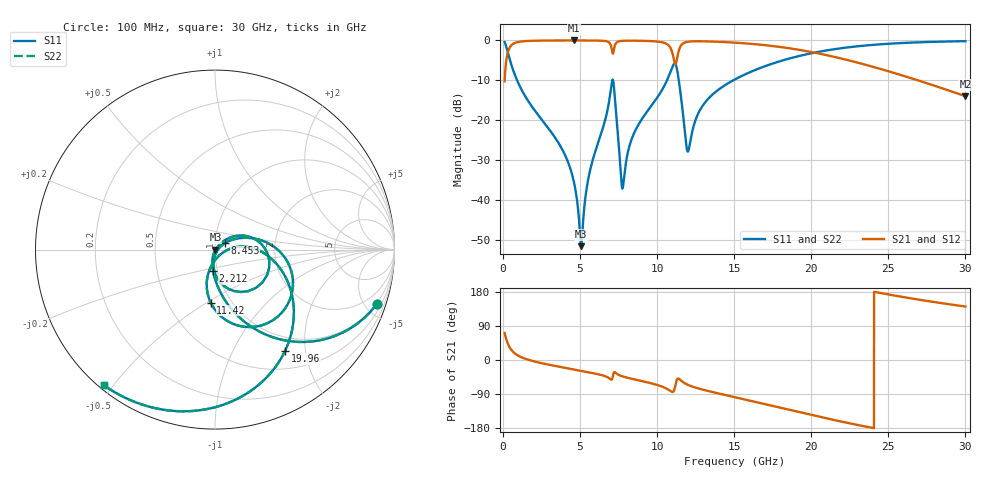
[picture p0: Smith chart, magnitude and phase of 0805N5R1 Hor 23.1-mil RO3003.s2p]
# GHz S MA R 50
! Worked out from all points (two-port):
!   3201 points, 100 MHz to 30 GHz, reference 50 ohm
!   highest |S21| = -0.02 dB at 4.594 GHz (marker M1); lowest = -14.0 dB at 30 GHz (marker M2)
!   |S21| within 3 dB of the highest: 307.7 MHz to 7.094 GHz (6.786 GHz wide, 183 % of centre); 11.37 GHz to 20.14 GHz (8.769 GHz wide, 55.7 % of centre)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
!   lowest |S11| = -51.5 dB at 5.071 GHz (marker M3), VSWR 1.01, Z = 50.2 - j0.12 ohm
!   |S11| at or under -10 dB: 908.1 MHz to 7.086 GHz (6.178 GHz wide, 155 % of centre); 7.138 GHz to 10.64 GHz (3.499 GHz wide, 39.4 % of centre); 11.4 GHz to 14.94 GHz (3.533 GHz wide, 26.8 % of centre)
!   |S22| runs from -51.5 to -0.2 dB; largest |S21 - S12| = 0
!   S11 on the Smith chart (normalised r, x): 100 MHz: 0.94, -6.00; 2.212 GHz: 0.95, -0.23; 8.453 GHz: 1.11, +0.08; 11.42 GHz: 0.80, -0.52; 19.96 GHz: 0.77, -1.64; 30 GHz: 0.01, -0.47
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0.1  0.9513 -18.5  0.3079 71.5  0.3079 71.5  0.9513 -18.5
0.7260313  0.3873 -71.2  0.9212 18.6  0.9212 18.6  0.3873 -71.2
2.211688  0.1209 -95.0  0.9912 -5.6  0.9912 -5.6  0.1209 -95.0
3.828156  0.04354 -106.6  0.9969 -19.2  0.9969 -19.2  0.04354 -106.6
4.594344  0.01699 -107.1  0.9974 -25.0  0.9974 -25.0  0.01699 -107.1
5.070875  0.002654 -26.8  0.9972 -28.6  0.9972 -28.6  0.002654 -26.8
5.089563  0.002778 -12.5  0.9971 -28.7  0.9971 -28.7  0.002778 -12.5
5.594125  0.02126 48.5  0.9963 -32.6  0.9963 -32.6  0.02126 48.5
7.061094  0.3005 -7.4  0.7618 -51.5  0.7618 -51.5  0.3005 -7.4
7.229281  0.2192 -73.8  0.826 -31.9  0.826 -31.9  0.2192 -73.8
7.743188  0.01395 -32.9  0.986 -43.2  0.986 -43.2  0.01395 -32.9
8.453312  0.06567 33.2  0.9904 -50.5  0.9904 -50.5  0.06567 33.2
10.06978  0.201 18.9  0.9638 -66.7  0.9638 -66.7  0.201 18.9
10.99481  0.4708 -22.6  0.6862 -84.3  0.6862 -84.3  0.4708 -22.6
11.42463  0.2966 -94.6  0.7668 -49.9  0.7668 -49.9  0.2966 -94.6
12.01328  0.04098 -40.5  0.9624 -65.9  0.9624 -65.9  0.04098 -40.5
12.96634  0.1535 6.4  0.9736 -78.3  0.9736 -78.3  0.1535 6.4
15.05  0.3249 -9.9  0.9363 -98.4  0.9363 -98.4  0.3249 -9.9
19.95547  0.6864 -55.3  0.7174 -144.6  0.7174 -144.6  0.6864 -55.3
20.03956  0.6917 -56.1  0.7123 -145.4  0.7123 -145.4  0.6917 -56.1
25.01978  0.9072 -97.7  0.4098 172.8  0.4098 172.8  0.9072 -97.7
30  0.9769 -129.4  0.2 141.1  0.2 141.1  0.9769 -129.4
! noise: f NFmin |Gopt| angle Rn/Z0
0.1  0.0007898  0.9225  1.156  0.002255
3.417  0.006031  0.6925  19.6  0.003715
6.743  0.0282  0.8605  37.6  0.03884
10.06  0.02921  0.8106  54.82  0.02541
13.39  0.02914  0.7624  71.12  0.01662
16.7  0.02897  0.72  85.36  0.01133
20.03  0.0358  0.7372  98.87  0.01188
23.35  0.04653  0.7715  111.8  0.01352
26.67  0.06312  0.8149  124.6  0.016
30  0.09031  0.8617  137.3  0.01922
